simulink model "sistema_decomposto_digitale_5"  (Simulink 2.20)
settings: Solver=VariableStepDiscrete  StartTime=0.0  StopTime=7.0  RelTol=1e-3  AbsTol=1e-6
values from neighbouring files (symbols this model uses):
  q0 = K*(1+Kbeta)    [pidin.m]
  q1 = -K*(delta+Kgamma-delta*Kalfa+Kbeta+delta*Kbeta)    [pidin.m]
  q2 = K*delta*(Kgamma-Kalfa*Kgamma+Kbeta)    [pidin.m]
  r1 = Kgamma+delta    [pidin.m]
  r2 = Kgamma*delta    [pidin.m]
undefined symbols (not defined in the file or in its folder): T

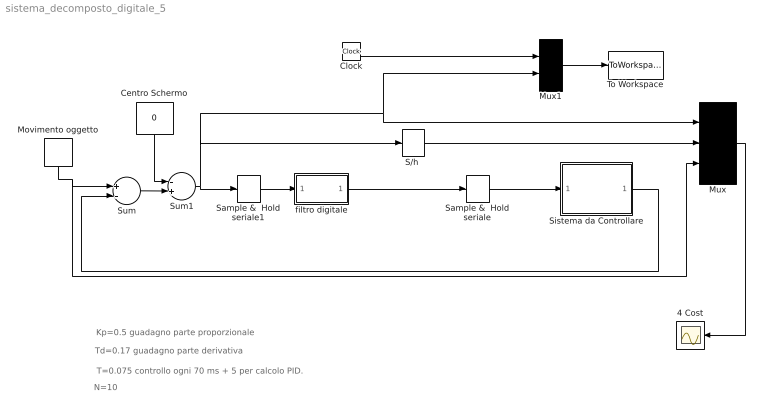
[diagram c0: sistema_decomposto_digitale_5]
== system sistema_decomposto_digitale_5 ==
  note: Kp=0.5 guadagno parte proporzionale
  note: Td=0.17 guadagno parte derivativa
  note: T=0.075 controllo ogni 70 ms + 5 per calcolo PID.
  note: N=10
  4 Cost : Scope
  Centro Schermo : Constant  Orientation=down  Value=0
  Clock : Clock
  Movimento oggetto : DiscretePulseGenerator  Orientation=down  Amplitude=45  Period=100  PulseWidth=100  PhaseDelay=1  SampleTime=.1
  Mux : Mux  Inputs=3
  Mux1 : Mux  Inputs=2
  "S/h " : ZeroOrderHold  SampleTime=.260
  Sample &  Hold seriale : ZeroOrderHold  SampleTime=.260
  Sample &  Hold seriale1 : ZeroOrderHold  SampleTime=T
  Sistema da Controllare : Subsystem
  Sum : Sum  Inputs=+-
  Sum1 : Sum  Inputs=-+
  To Workspace : ToWorkspace  VariableName=sim  SampleTime=.01
  filtro digitale : Subsystem
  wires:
  Sum/1 -> Sum1/2
  Centro Schermo/1 -> Sum1/1
  Sum1/1 -> "S/h "/1, Mux/1, Mux1/2, Sample &  Hold seriale1/1
  Movimento oggetto/1 -> Sum/1, Mux/3
  filtro digitale/1(Out1) -> Sample &  Hold seriale/1
  Sample &  Hold seriale/1 -> Sistema da Controllare/1(In1)
  "S/h "/1 -> Mux/2
  Sample &  Hold seriale1/1 -> filtro digitale/1(In1)
  Mux/1 -> 4 Cost/1
  Sistema da Controllare/1(Out1) -> Sum/2
  Mux1/1 -> To Workspace/1
  Clock/1 -> Mux1/1

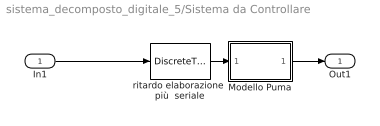
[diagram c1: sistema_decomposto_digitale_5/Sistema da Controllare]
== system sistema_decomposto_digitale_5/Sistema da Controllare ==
  In1 : Inport  Port=1  PortWidth=-1  SampleTime=-1
  Modello Puma : Subsystem  Description=Modello Puma
  ritardo elaborazione  più  seriale : DiscreteTransferFcn  Numerator=1  Denominator=[1 0 0 0 0 0 0 0 0]  SampleTime=.032
  Out1 : Outport  Port=1
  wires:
  ritardo elaborazione  più  seriale/1 -> Modello Puma/1(In1)
  Modello Puma/1(Out1) -> Out1/1
  In1/1 -> ritardo elaborazione  più  seriale/1

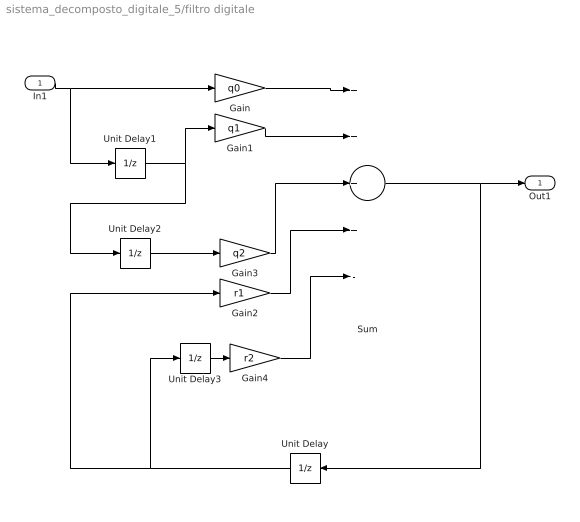
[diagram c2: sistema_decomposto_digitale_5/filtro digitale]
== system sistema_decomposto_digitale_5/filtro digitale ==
  In1 : Inport  Port=1  PortWidth=-1  SampleTime=-1
  Gain : Gain  Gain=q0
  Gain1 : Gain  Gain=q1
  Gain2 : Gain  Gain=r1
  Gain3 : Gain  Gain=q2
  Gain4 : Gain  Gain=r2
  Sum : Sum  Inputs=++++-
  Unit Delay : UnitDelay  Orientation=left  X0=0  SampleTime=T
  Unit Delay1 : UnitDelay  X0=0  SampleTime=T
  Unit Delay2 : UnitDelay  X0=0  SampleTime=T
  Unit Delay3 : UnitDelay  X0=0  SampleTime=T
  Out1 : Outport  Port=1
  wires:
  Gain1/1 -> Sum/2
  Gain/1 -> Sum/1
  In1/1 -> Gain/1, Unit Delay1/1
  Sum/1 -> Unit Delay/1, Out1/1
  Unit Delay1/1 -> Gain1/1, Unit Delay2/1
  Unit Delay2/1 -> Gain3/1
  Gain3/1 -> Sum/3
  Gain2/1 -> Sum/4
  Unit Delay/1 -> Gain2/1, Unit Delay3/1
  Unit Delay3/1 -> Gain4/1
  Gain4/1 -> Sum/5

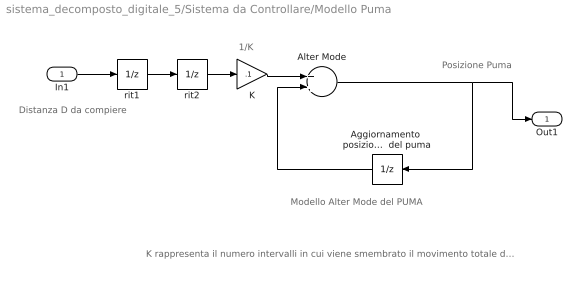
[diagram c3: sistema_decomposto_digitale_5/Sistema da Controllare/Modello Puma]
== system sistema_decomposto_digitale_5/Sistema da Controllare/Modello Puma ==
  note: Posizione Puma
  note: Modello Alter Mode del PUMA
  note: 1/K
  note: K rappresenta il numero intervalli in cui viene smembrato il movimento totale da compiere, dopo K time-slice (del PUMA) si ottiene che si e' compiuto proprio la distanza D trasmessa.
  note: Distanza D da compiere
  In1 : Inport  Port=1  PortWidth=-1  SampleTime=-1
  Aggiornamento  posizione   Il sample-time di questo blocco rappresenta la TIME-SLICE  del puma : UnitDelay  Orientation=left  X0=0  SampleTime=.032
  Alter Mode : Sum  Inputs=++
  K : Gain  Gain=.1
  rit1 : UnitDelay  X0=0  SampleTime=.032
  rit2 : UnitDelay  X0=0  SampleTime=.032
  Out1 : Outport  Port=1
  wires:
  K/1 -> Alter Mode/1
  Aggiornamento  posizione   Il sample-time di questo blocco rappresenta la TIME-SLICE  del puma/1 -> Alter Mode/2
  Alter Mode/1 -> Out1/1, Aggiornamento  posizione   Il sample-time di questo blocco rappresenta la TIME-SLICE  del puma/1
  In1/1 -> rit1/1
  rit1/1 -> rit2/1
  rit2/1 -> K/1
